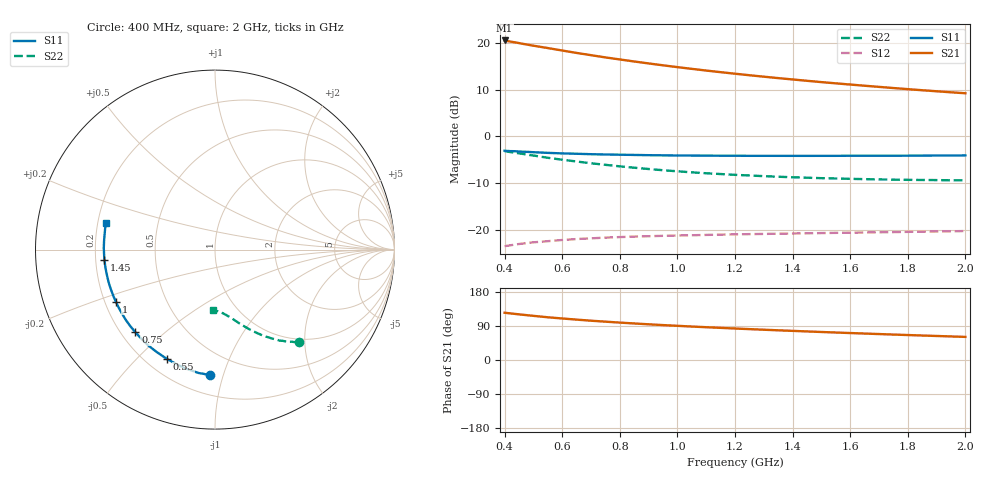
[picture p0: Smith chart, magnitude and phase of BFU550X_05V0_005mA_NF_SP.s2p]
! Filename:  P:\Prog\Test\Noise\ATS_data\Testdata_Net\BFU550X no attenuator noise\BFU550X_APG2013_44_C05_05p0V_005mA_NF_CM01_D.sf
! Date/Time: Fri 26/Jul/2013 14:37:12
! BFU550X_APG2013_44_C05_05p0V_1to10mA_NF_CM01_Bias4_R.sf
! Noise Parameter Data File
! BFU550X_APG2013_44_C05_05p0V_1to10mA_NF_CM01
! Date/time: Wed Jul 24 16:36:15 2013
! VAR V_out= 5.000000
! VAR I_out= 5.000000
! VAR V_in= 0.812400
! VAR I_in= 0.054910
! Device data file deembeded for feedlines and parallel
! Original file: \BFU550X no attenuator noise\BFU550X_APG2013_44_C05_05p0V_005mA_NF_CM01_R.sf
! Feed-files: PR005V01_100713_Feed1.s2p, PR005V01_100713_Feed2.s2p
! Parallel-file: PR005V01_100713_Par.s2p
# MHz S MA R 50
!  Freq-MHz  S11-mag  S11-arg  S21-mag  S21-arg  S12-mag  S12-arg  S22-mag  S22-arg
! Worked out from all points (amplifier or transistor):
!   37 points, 400 MHz to 2 GHz, reference 50 ohm
!   highest |S21| = 20.5 dB at 400 MHz (marker M1)
!   |S21| within 3 dB of that: start of sweep to 684.2 MHz
!   unconditionally stable (mu >= 1): nowhere
!   at 500 MHz: K = 0.27, MSG = 21.1 dB, |S12| = -22.7 dB
!   at 1.1 GHz: K = 0.56, MSG = 17.6 dB, |S12| = -21.1 dB
!   at 2 GHz: K = 0.90, MSG = 14.8 dB, |S12| = -20.3 dB
!   lowest NFmin = 0.64 dB at 460 MHz
!   S11 on the Smith chart (normalised r, x): 400 MHz: 0.33, -0.91; 550 MHz: 0.28, -0.62; 750 MHz: 0.26, -0.40; 1 GHz: 0.24, -0.23; 1.45 GHz: 0.24, -0.04; 2 GHz: 0.23, +0.12
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400  0.7012 -92.3  10.64 124.7  0.06667 46.2  0.6957 -47.9
420  0.6948 -95.3  10.35 123.0  0.06811 45.1  0.678 -49.4
440  0.6913 -98.5  10.11 121.3  0.06968 44.0  0.6645 -50.6
460  0.6854 -101.3  9.833 119.6  0.07096 42.8  0.6509 -52.1
500  0.6764 -107.0  9.357 116.5  0.07332 40.8  0.6234 -54.5
550  0.6657 -113.7  8.826 112.8  0.0754 38.7  0.5895 -57.2
600  0.6568 -119.3  8.306 109.5  0.07765 36.9  0.5623 -59.6
650  0.6511 -124.6  7.827 106.5  0.07949 35.3  0.5379 -61.8
700  0.6442 -129.6  7.404 103.7  0.08089 33.9  0.5149 -63.8
750  0.6396 -133.9  7.009 101.2  0.08231 32.8  0.4957 -65.5
800  0.6359 -138.2  6.662 98.7  0.08342 31.8  0.4773 -67.3
850  0.6325 -142.1  6.338 96.4  0.08446 30.9  0.4614 -68.8
900  0.6286 -145.8  6.04 94.2  0.08527 30.2  0.447 -70.2
950  0.6265 -149.2  5.767 92.1  0.08603 29.5  0.4338 -71.6
1000  0.6238 -152.3  5.514 90.2  0.08674 29.0  0.4224 -72.8
1100  0.6212 -158.1  5.067 86.5  0.088 28.2  0.4026 -75.2
1200  0.6199 -163.4  4.687 83.1  0.0892 27.6  0.3873 -77.4
1300  0.6188 -168.2  4.357 79.9  0.09018 27.3  0.375 -79.4
1450  0.6183 -174.8  3.936 75.4  0.09161 27.1  0.3607 -82.2
1500  0.6185 -176.8  3.81 73.9  0.09206 27.0  0.3567 -83.1
1750  0.6203 174.0  3.292 67.2  0.09432 27.4  0.3438 -87.5
2000  0.625 166.0  2.894 61.0  0.09684 28.3  0.3382 -91.5
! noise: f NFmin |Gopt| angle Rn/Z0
400  0.6893  0.1733  38.27  0.1122
460  0.6396  0.1448  69.96  0.0858
600  0.7336  0.1754  64.58  0.104
800  0.7379  0.1774  94.52  0.0849
1000  0.7707  0.2158  104.1  0.0854
1200  0.8029  0.2532  122.2  0.0759
1400  0.8498  0.2865  131.7  0.0726
1600  0.8666  0.3392  149.3  0.0541
1800  0.9273  0.3742  162  0.046
2000  0.9302  0.4183  169  0.0418
